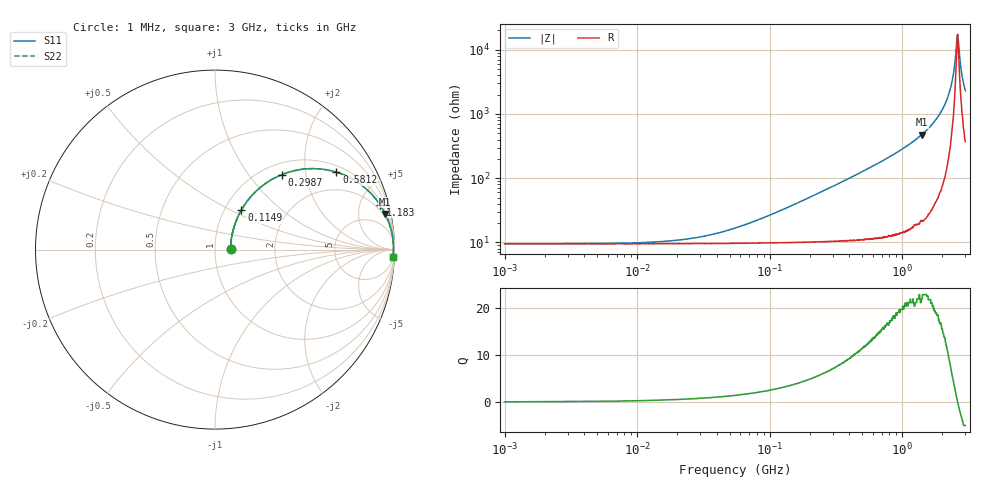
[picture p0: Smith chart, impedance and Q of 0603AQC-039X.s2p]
!s-Parameter Generated by FASTRON Sdn. Bhd.
!FASTRON P/N : 0603AQC-039X
!Keysight Technologies: E4991B_MY54100416_A.01.15
!Date: Thu Jun 25 13:54:00 2026
!Version  :Rev00  Thu Jun 25 13:54:00 2026
!Data & Calibration Information:
!Freq  S11  S21  S12  S22
!PortZ  Port1:50+j0  Port2:50+j0
!When reading reference impedance value at option line is always used.
! Remarks : This data is being provided solely for informational purposes.
# Hz S dB R 50
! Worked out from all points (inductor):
!   1601 points, 1 MHz to 3 GHz, reference 50 ohm
!   read as one part in series: L = 39 nH near 120.2 MHz
!   highest Q = 22.9 at 1.402 GHz (marker M1), where L = 53.8 nH
!   self-resonance near 2.608 GHz
!   S11 on the Smith chart (normalised r, x): 1 MHz: 1.19, +0.01; 114.9 MHz: 1.20, +0.57; 298.7 MHz: 1.21, +1.48; 581.2 MHz: 1.23, +2.97; 1.183 GHz: 1.34, +7.20; 3 GHz: 8, -45
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1000000  -21.20 1.4  -0.79 -0.1  -0.79 -0.1  -21.20 1.4
3804036  -21.20 5.5  -0.79 -0.5  -0.79 -0.5  -21.20 5.5
1.447069e7  -20.60 19.4  -0.80 -1.9  -0.80 -1.9  -20.60 19.4
2.801249e7  -19.30 32.7  -0.82 -3.7  -0.82 -3.7  -19.30 32.7
5.504702e7  -16.40 47.6  -0.87 -7.1  -0.87 -7.1  -16.40 47.6
1.148668e8  -11.50 56.3  -1.10 -14.5  -1.10 -14.5  -11.50 56.3
2.083556e8  -7.32 53.8  -1.69 -25.0  -1.69 -25.0  -7.32 53.8
2.987278e8  -5.02 48.2  -2.47 -33.8  -2.47 -33.8  -5.02 48.2
5.81181e8  -1.91 32.5  -5.37 -53.1  -5.37 -53.1  -1.91 32.5
7.925923e8  -1.07 24.6  -7.59 -61.9  -7.59 -61.9  -1.07 24.6
1.182785e9  -0.43 15.3  -11.60 -72.0  -11.60 -72.0  -0.43 15.3
1.402151e9  -0.27 11.8  -13.80 -75.6  -13.80 -75.6  -0.27 11.8
1.800756e9  -0.12 6.9  -18.40 -80.1  -18.40 -80.1  -0.12 6.9
2.145442e9  -0.06 3.6  -23.90 -81.6  -23.90 -81.6  -0.06 3.6
2.266846e9  -0.05 2.6  -26.70 -81.0  -26.70 -81.0  -0.05 2.6
2.371269e9  -0.05 1.8  -29.90 -78.7  -29.90 -78.7  -0.05 1.8
2.443543e9  -0.05 1.3  -32.80 -75.3  -32.80 -75.3  -0.05 1.3
2.543347e9  -0.05 0.5  -39.20 -58.9  -39.20 -58.9  -0.05 0.5
2.607784e9  -0.05 0.1  -44.60 -13.6  -44.60 -13.6  -0.05 0.1
2.673854e9  -0.05 -0.4  -41.30 46.7  -41.30 46.7  -0.05 -0.4
2.853575e9  -0.06 -1.5  -31.20 74.3  -31.20 74.3  -0.06 -1.5
3e9  -0.07 -2.4  -27.30 78.3  -27.30 78.3  -0.07 -2.4
